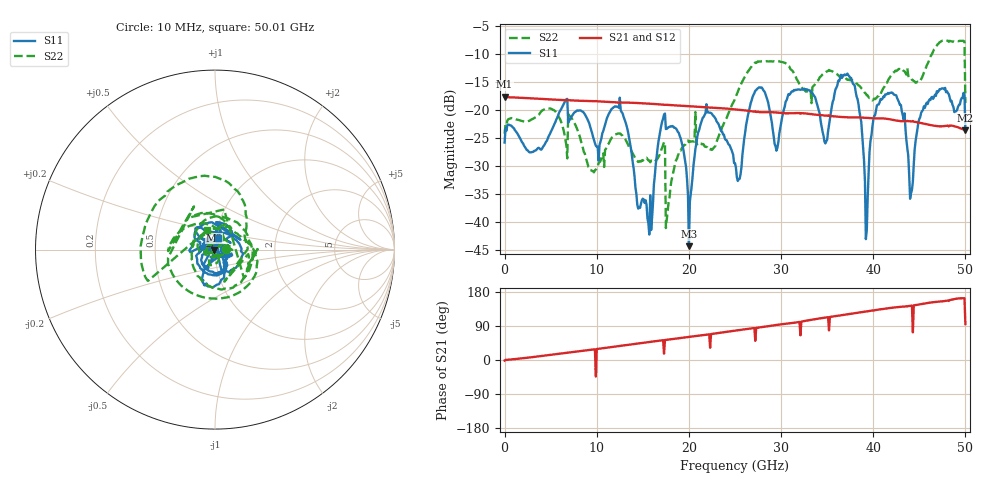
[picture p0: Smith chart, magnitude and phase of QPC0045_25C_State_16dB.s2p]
!File name = QPC0045_25C_State_16dB.s2p
!Date Time: 2024/05/02 05:42:16 AM
!Cal Ref Plane:TRL
!TEMP = 25C
!Vdd(V) = 3.15
!Vss(V) = 0.000
# GHz  S  DB  R  50
!%	Freq(GHz)  S11(dB)  S11(deg)  S21(dB)  S21(deg)  S12(dB)  S12(deg)  S22(dB)  S22(deg)
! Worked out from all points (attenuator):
!   501 points, 10 MHz to 50.01 GHz, reference 50 ohm
!   highest |S21| = -17.58 dB at 10 MHz (marker M1); lowest = -23.6 dB at 50.01 GHz (marker M2)
!   lowest |S11| = -44.3 dB at 20.01 GHz (marker M3), VSWR 1.01, Z = 49.4 - j0.215 ohm
!   |S11| at or under -10 dB: start of sweep to end of sweep
!   |S22| runs from -41.0 to -7.5 dB; largest |S21 - S12| = 0.00045
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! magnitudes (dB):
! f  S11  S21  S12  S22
! 10 MHz  -25.8  -17.6  -17.6  -24.2
! 8.41 GHz  -20.2  -18.3  -18.3  -26.1
! 10.11 GHz  -26.5  -18.4  -18.4  -30.0
! 12.61 GHz  -20.0  -18.6  -18.6  -24.2
! 15.71 GHz  -42.2  -18.8  -18.8  -29.0
! 16.71 GHz  -25.5  -18.9  -18.9  -28.3
! 17.71 GHz  -23.2  -19.0  -19.0  -37.9
! 20.01 GHz  -44.3  -19.3  -19.3  -25.7
! 21.91 GHz  -18.9  -19.5  -19.5  -26.5
! 25.01 GHz  -29.5  -19.8  -19.8  -17.9
! 27.41 GHz  -16.2  -20.3  -20.3  -11.4
! 29.51 GHz  -27.2  -20.4  -20.4  -11.2
! 33.41 GHz  -16.9  -20.7  -20.7  -15.9
! 34.81 GHz  -25.9  -20.9  -20.9  -13.2
! 37.81 GHz  -15.3  -21.3  -21.3  -14.7
! 39.31 GHz  -41.4  -21.3  -21.3  -17.3
! 40.11 GHz  -21.0  -21.4  -21.4  -17.9
! 41.71 GHz  -17.0  -21.6  -21.6  -14.3
! 43.21 GHz  -20.9  -21.9  -21.9  -12.8
! 44.11 GHz  -34.8  -22.0  -22.0  -14.3
! 45.91 GHz  -18.9  -22.5  -22.5  -11.7
! 50.01 GHz  -23.4  -23.6  -23.5  -18.7
